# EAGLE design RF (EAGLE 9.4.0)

## Sheet 1 of 3: Board to Board Headers
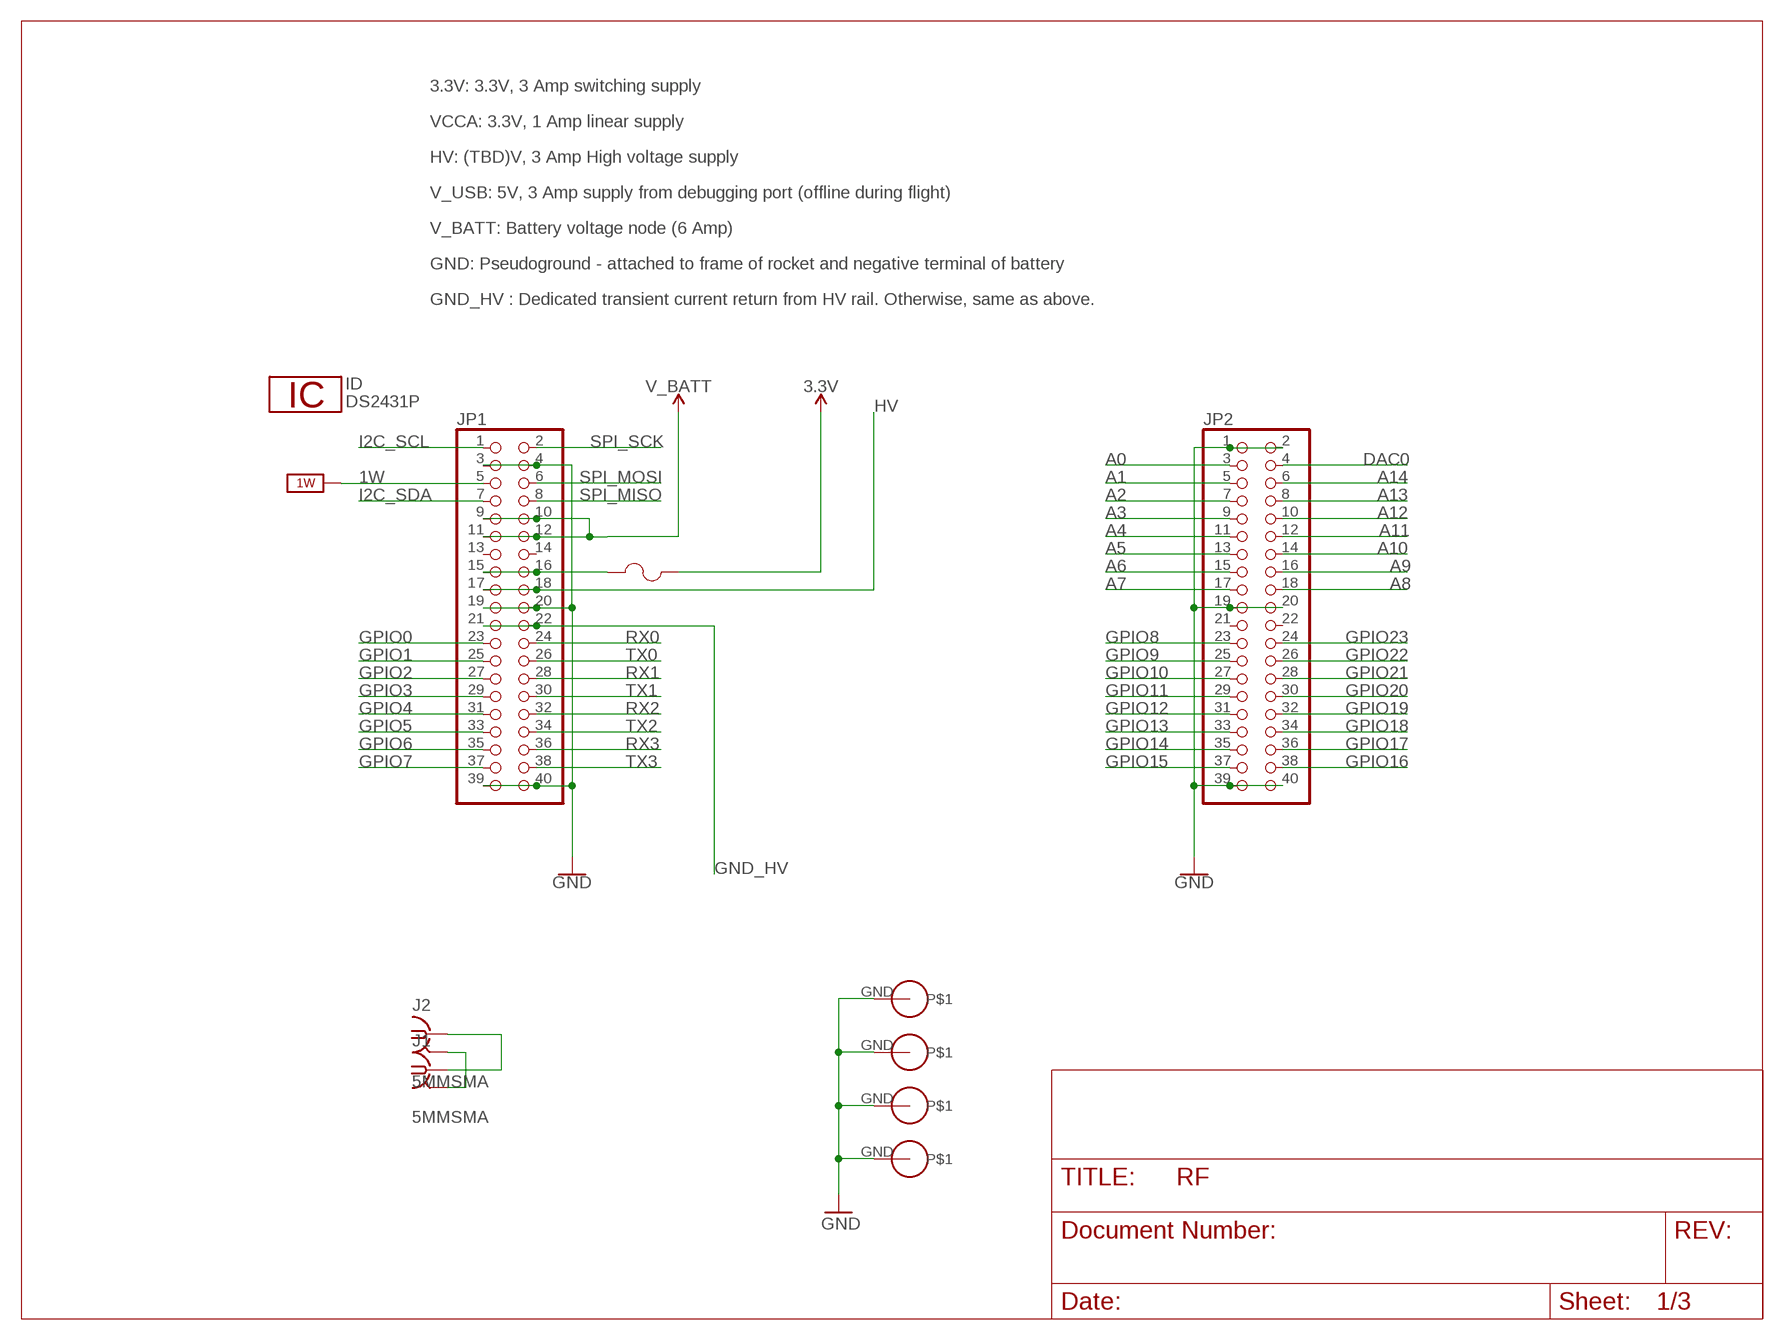
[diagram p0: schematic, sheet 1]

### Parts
F1  0603SFF150F/32-2  [FUS0603_TYCO]
ID  DS2431P  [TSOC6]
J1  5MMSMA  [5MMSMA]
J2  5MMSMA  [5MMSMA]
JP1  PINHD-2X20  [2X20]
JP2  PINHD-2X20  [2X20]
U$1  PS/104-MOUNTING-HOLE  [PC/104-MOUNTING-HOLE]
U$2  PS/104-MOUNTING-HOLE  [PC/104-MOUNTING-HOLE]
U$3  PS/104-MOUNTING-HOLE  [PC/104-MOUNTING-HOLE]
U$4  PS/104-MOUNTING-HOLE  [PC/104-MOUNTING-HOLE]

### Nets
1W: JP1.5 ; supply symbol labelled 1W_SUP
3.3V: F1.2 ; also sheet 2
A0: JP2.3
A1: JP2.5
A2: JP2.7
A3: JP2.9
A4: JP2.11
A5: JP2.13
A6: JP2.15
A7: JP2.17
A8: JP2.18
A9: JP2.16
A10: JP2.14
A11: JP2.12
A12: JP2.10
A13: JP2.8
A14: JP2.6
DAC0: JP2.4
GND: J1.GND J1.GND2(GND) J2.GND J2.GND2(GND) JP1.3 JP1.4 JP1.19 JP1.20 JP1.39 JP1.40 JP2.1 JP2.2 JP2.19 JP2.20 JP2.39 JP2.40 U$1.GND U$2.GND U$3.GND U$4.GND ; also sheet 2
GND_HV: JP1.21 JP1.22
GPIO0: JP1.23
GPIO1: JP1.25
GPIO2: JP1.27
GPIO3: JP1.29
GPIO4: JP1.31
GPIO5: JP1.33
GPIO6: JP1.35
GPIO7: JP1.37
GPIO8: JP2.23
GPIO9: JP2.25
GPIO10: JP2.27
GPIO11: JP2.29
GPIO12: JP2.31
GPIO13: JP2.33
GPIO14: JP2.35
GPIO15: JP2.37
GPIO16: JP2.38
GPIO17: JP2.36
GPIO18: JP2.34
GPIO19: JP2.32
GPIO20: JP2.30
GPIO21: JP2.28
GPIO22: JP2.26
GPIO23: JP2.24
HV: JP1.17 JP1.18
I2C_SCL: JP1.1
I2C_SDA: JP1.7
N$3: F1.1 JP1.15 JP1.16
N$4: JP1.9 JP1.10 JP1.11 JP1.12
N$8: J1.RF J2.RF
RX0: JP1.24 ; also sheet 2
RX1: JP1.28 ; also sheet 2
RX2: JP1.32 ; also sheet 2
RX3: JP1.36
SPI_MISO: JP1.8
SPI_MOSI: JP1.6
SPI_SCK: JP1.2
TX0: JP1.26 ; also sheet 2
TX1: JP1.30 ; also sheet 2
TX2: JP1.34 ; also sheet 2
TX3: JP1.38
Unconnected: JP1.13 JP1.14 JP2.21 JP2.22

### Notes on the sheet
- 3.3V: 3.3V, 3 Amp switching supply
- VCCA: 3.3V, 1 Amp linear supply
- HV: (TBD)V, 3 Amp High voltage supply
- V_USB: 5V, 3 Amp supply from debugging port (offline during flight)
- V_BATT: Battery voltage node (6 Amp)
- GND: Pseudoground - attached to frame of rocket and negative terminal of battery
- GND_HV : Dedicated transient current return from HV rail. Otherwise, same as above.

## Sheet 2 of 3: RN2483 434MHz RF module
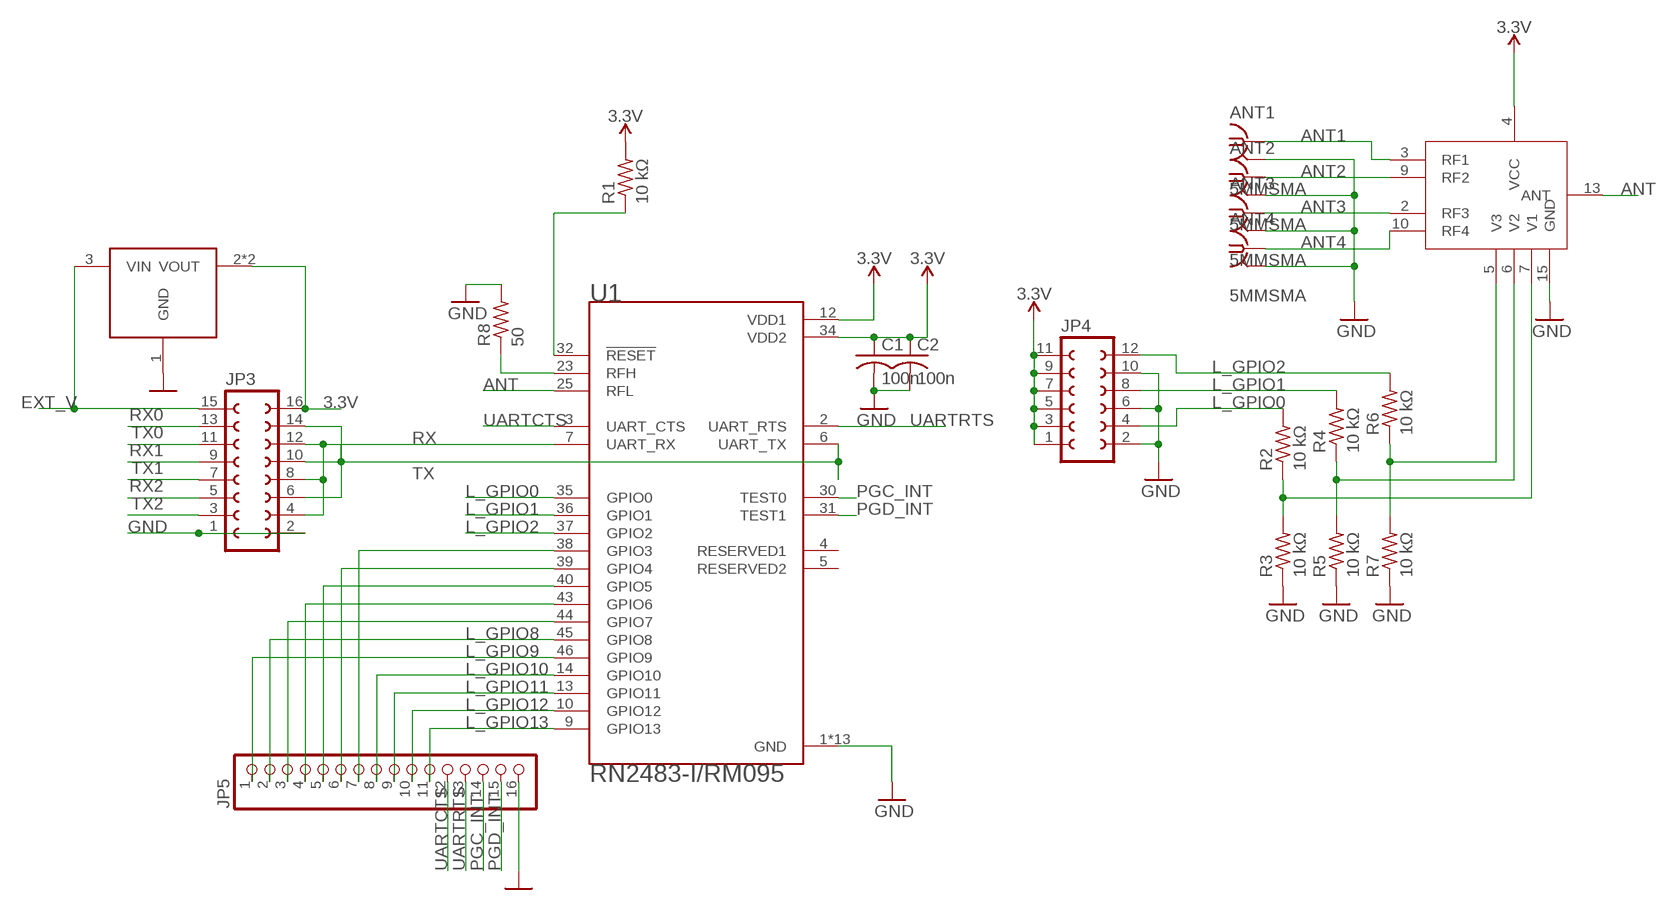
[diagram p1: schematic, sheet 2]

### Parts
ANT1  5MMSMA  [5MMSMA]
ANT2  5MMSMA  [5MMSMA]
ANT3  5MMSMA  [5MMSMA]
ANT4  5MMSMA  [5MMSMA]
C1  100n  C-USC0805  [C0805]
C2  100n  C-USC0805  [C0805]
JP3  FE08-2  [FE08-2]
JP4  FE06-2  [FE06-2]
JP5  PINHD-1X16  [1X16]
R1  10 kΩ  R-US_R1206  [R1206]
R2  10 kΩ  R-US_R1206  [R1206]
R3  10 kΩ  R-US_R1206  [R1206]
R4  10 kΩ  R-US_R1206  [R1206]
R5  10 kΩ  R-US_R1206  [R1206]
R6  10 kΩ  R-US_R1206  [R1206]
R7  10 kΩ  R-US_R1206  [R1206]
R8  50  R-US_R1206  [R1206]
U1  RN2483-I/RM095  [MICROCHIP_RN2483-I/RM095]
U2  SKY13414  [QFN45P200X200X55-15N]
U3  LDL1117S33R  [SOT223]

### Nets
3.3V: C1.1 C2.1 JP3.16 JP4.1 JP4.3 JP4.5 JP4.7 JP4.9 JP4.11 R1.2 U1.12(VDD1) U1.34(VDD2) U2.4(VCC) U3.2(VOUT) U3.4(VOUT) ; also sheet 1
ANT: U1.25(RFL) U2.13(ANT)
ANT1: ANT1.RF U2.3(RF1)
ANT2: ANT2.RF U2.9(RF2)
ANT3: ANT3.RF U2.2(RF3)
ANT4: ANT4.RF U2.10(RF4)
EXT_V: JP3.15 U3.3(VIN)
GND: ANT1.GND ANT1.GND2(GND) ANT2.GND ANT2.GND2(GND) ANT3.GND ANT3.GND2(GND) ANT4.GND ANT4.GND2(GND) C1.2 C2.2 JP3.1 JP3.2 JP4.2 JP4.6 JP4.10 JP5.16 R3.1 R5.1 R7.1 R8.2 U1.1(GND) U1.8(GND) U1.11(GND) U1.20(GND) U1.21(GND) U1.22(GND) U1.24(GND) U1.26(GND) U1.27(GND) U1.28(GND) U1.33(GND) U1.41(GND) U1.47(GND) U2.15(GND) U3.1(GND) ; also sheet 1
L_GPIO0: JP4.4 R2.2 U1.35(GPIO0)
L_GPIO1: JP4.8 R4.2 U1.36(GPIO1)
L_GPIO2: JP4.12 R6.2 U1.37(GPIO2)
L_GPIO8: JP5.2 U1.45(GPIO8)
L_GPIO9: JP5.1 U1.46(GPIO9)
L_GPIO10: JP5.8 U1.14(GPIO10)
L_GPIO11: JP5.9 U1.13(GPIO11)
L_GPIO12: JP5.10 U1.10(GPIO12)
L_GPIO13: JP5.11 U1.9(GPIO13)
N$1: R2.1 R3.2 U2.7(V1)
N$2: R4.1 R5.2 U2.6(V2)
N$7: R6.1 R7.2 U2.5(V3)
N$9: R1.1 U1.32(!RESET)
N$10: R8.1 U1.23(RFH)
N$16: JP5.3 U1.44(GPIO7)
N$17: JP5.4 U1.43(GPIO6)
N$18: JP5.5 U1.40(GPIO5)
N$19: JP5.6 U1.39(GPIO4)
N$20: JP5.7 U1.38(GPIO3)
PGC_INT: JP5.14 U1.30(TEST0)
PGD_INT: JP5.15 U1.31(TEST1)
RX: JP3.6 JP3.10 JP3.14 U1.6(UART_TX)
RX0: JP3.13 ; also sheet 1
RX1: JP3.9 ; also sheet 1
RX2: JP3.5 ; also sheet 1
TX: JP3.4 JP3.8 JP3.12 U1.7(UART_RX)
TX0: JP3.11 ; also sheet 1
TX1: JP3.7 ; also sheet 1
TX2: JP3.3 ; also sheet 1
UARTCTS: JP5.12 U1.3(UART_CTS)
UARTRTS: JP5.13 U1.2(UART_RTS)
Unconnected: U1.4(RESERVED1) U1.5(RESERVED2)

## Sheet 3 of 3: RN2903 903MHz RF module

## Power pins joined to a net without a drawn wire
1W: ID.2(1W)
GND: ID.1(GND)

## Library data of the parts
ANT1-ANT4 J1 J2 = CUINSPACE_Managed:5MMSMA
C1 C2 = rcl:C-US: CAPACITOR, American symbol; SPICEPREFIX: C
F1 = CU inSpace 2019 Parts:0603SFF150F/32-2; MANUFACTURER_PART_NUMBER: 0603SFF150F322; VENDOR: Littelfuse Inc
ID = 1wire:DS2431: 1024-Bit EEPROM
JP1 JP2 = pinhead:PINHD-2X20: PIN HEADER
JP3 = con-lsta:FE08-2: FEMALE HEADER; OC_FARNELL: unknown; OC_NEWARK: unknown
JP4 = con-lsta:FE06-2: FEMALE HEADER; OC_FARNELL: unknown; OC_NEWARK: unknown
JP5 = pinhead:PINHD-1X16: PIN HEADER
R1-R8 = rcl:R-US_: RESISTOR, American symbol; SPICEPREFIX: R
U1 = RN2483-I_RM095:RN2483-I/RM095: Sub-GHz Dual Band Long Range Transceiver LoRa Module; AVAILABILITY: Unavailable; DESCRIPTION: Sub-GHz Dual Band Long Range Transceiver LoRa Module; MF: Microchip; MP: RN2483-I/RM095; PACKAGE: None; PRICE: None
U2 = CUINSPACE_Managed:SKY13414
U3 = CUINSPACE_Managed:LDL1117S33R
U$1-U$4 = CU inSpace 2019 Parts:PS/104-MOUNTING-HOLE: Mounting hole for PC/104 board.

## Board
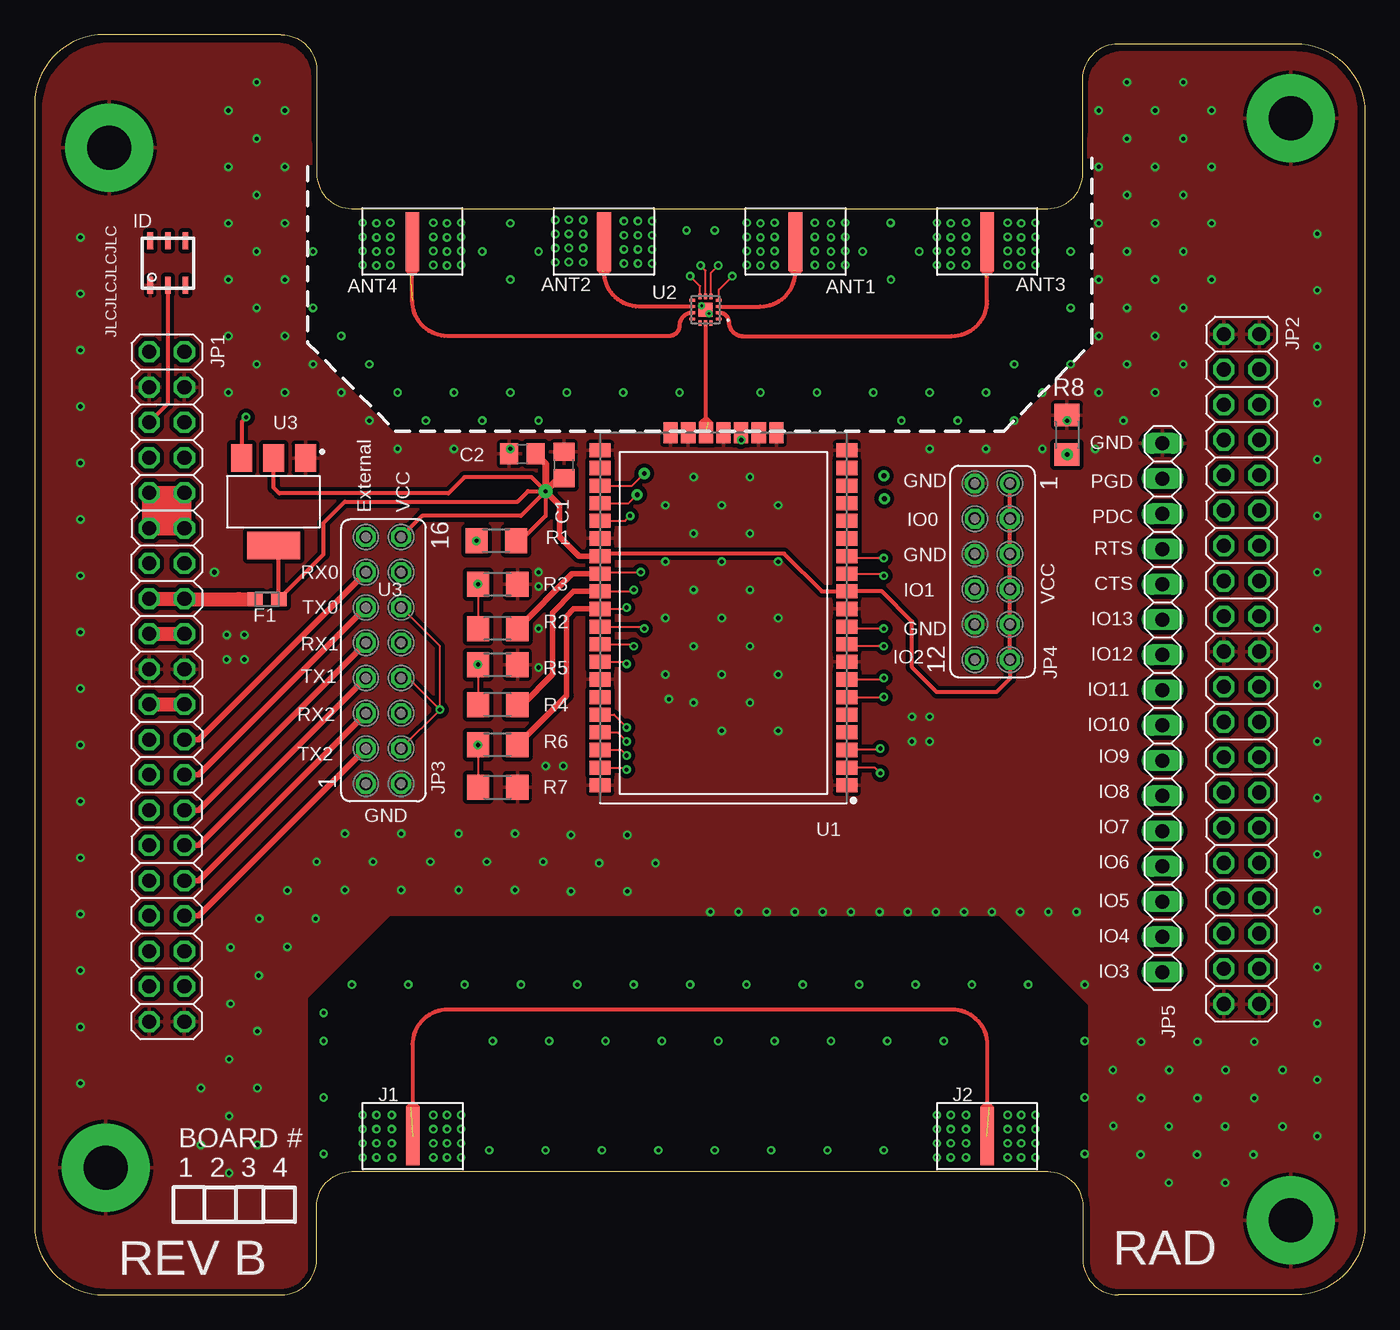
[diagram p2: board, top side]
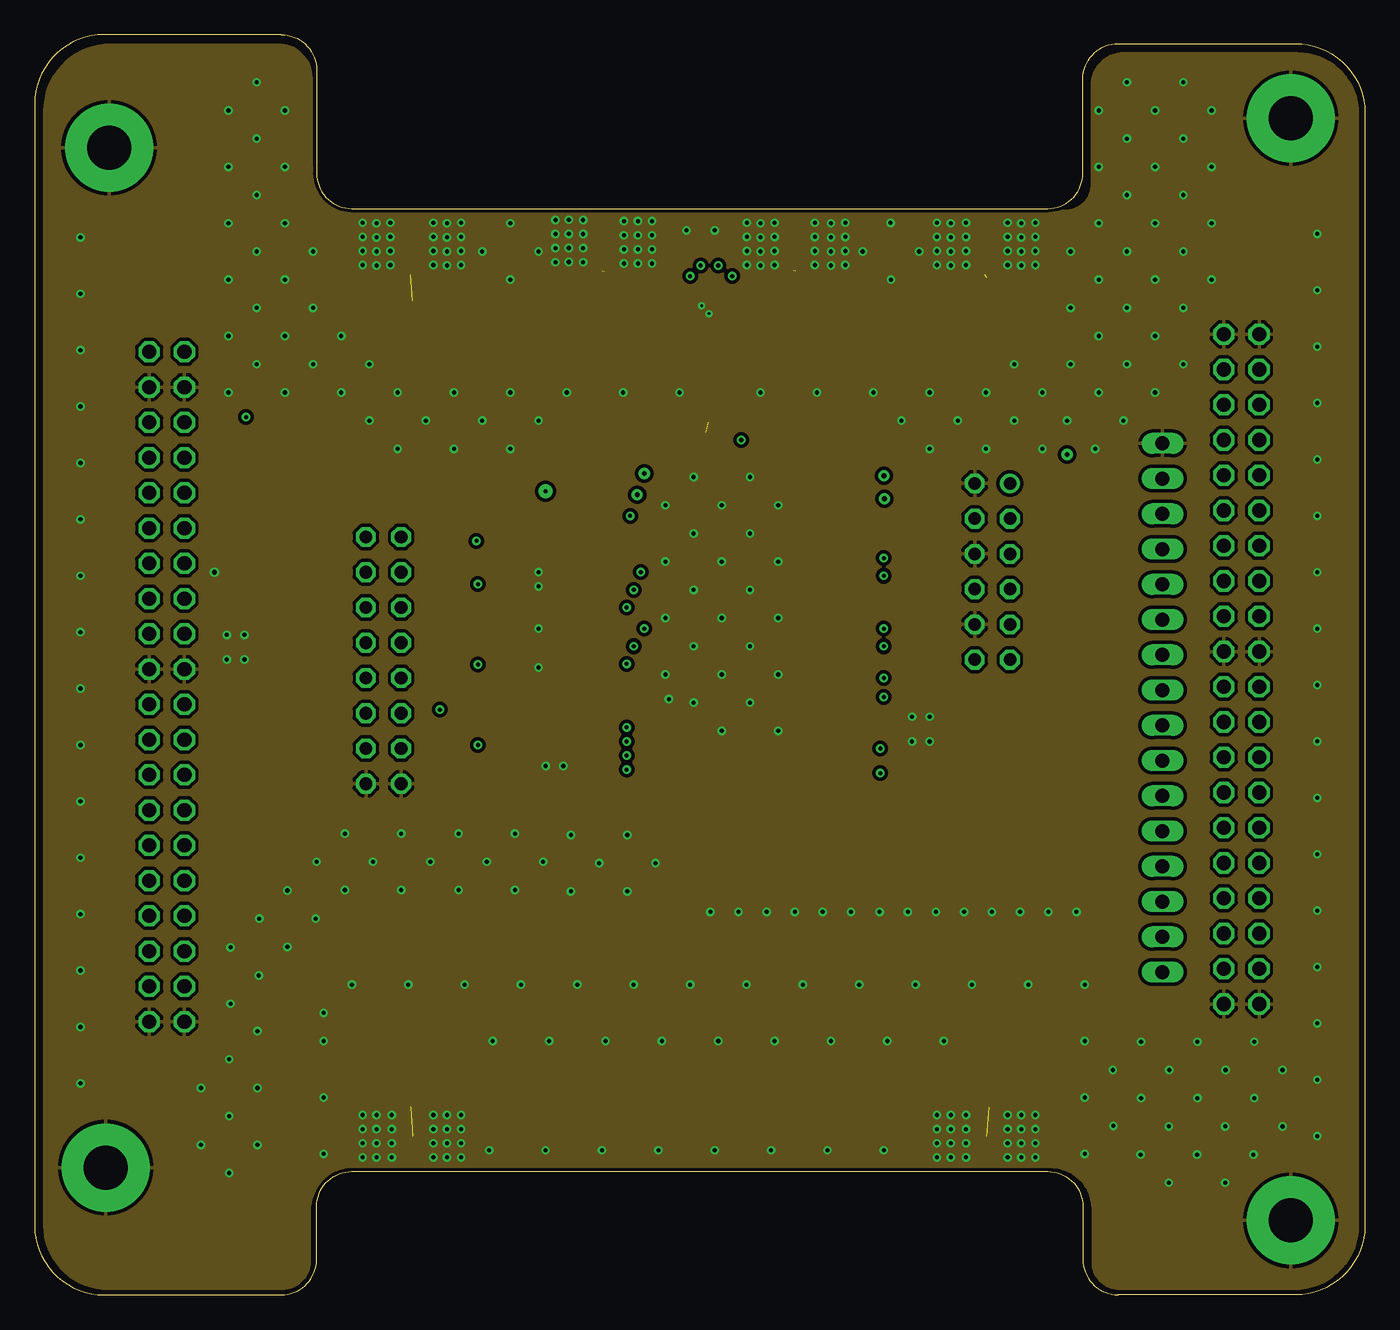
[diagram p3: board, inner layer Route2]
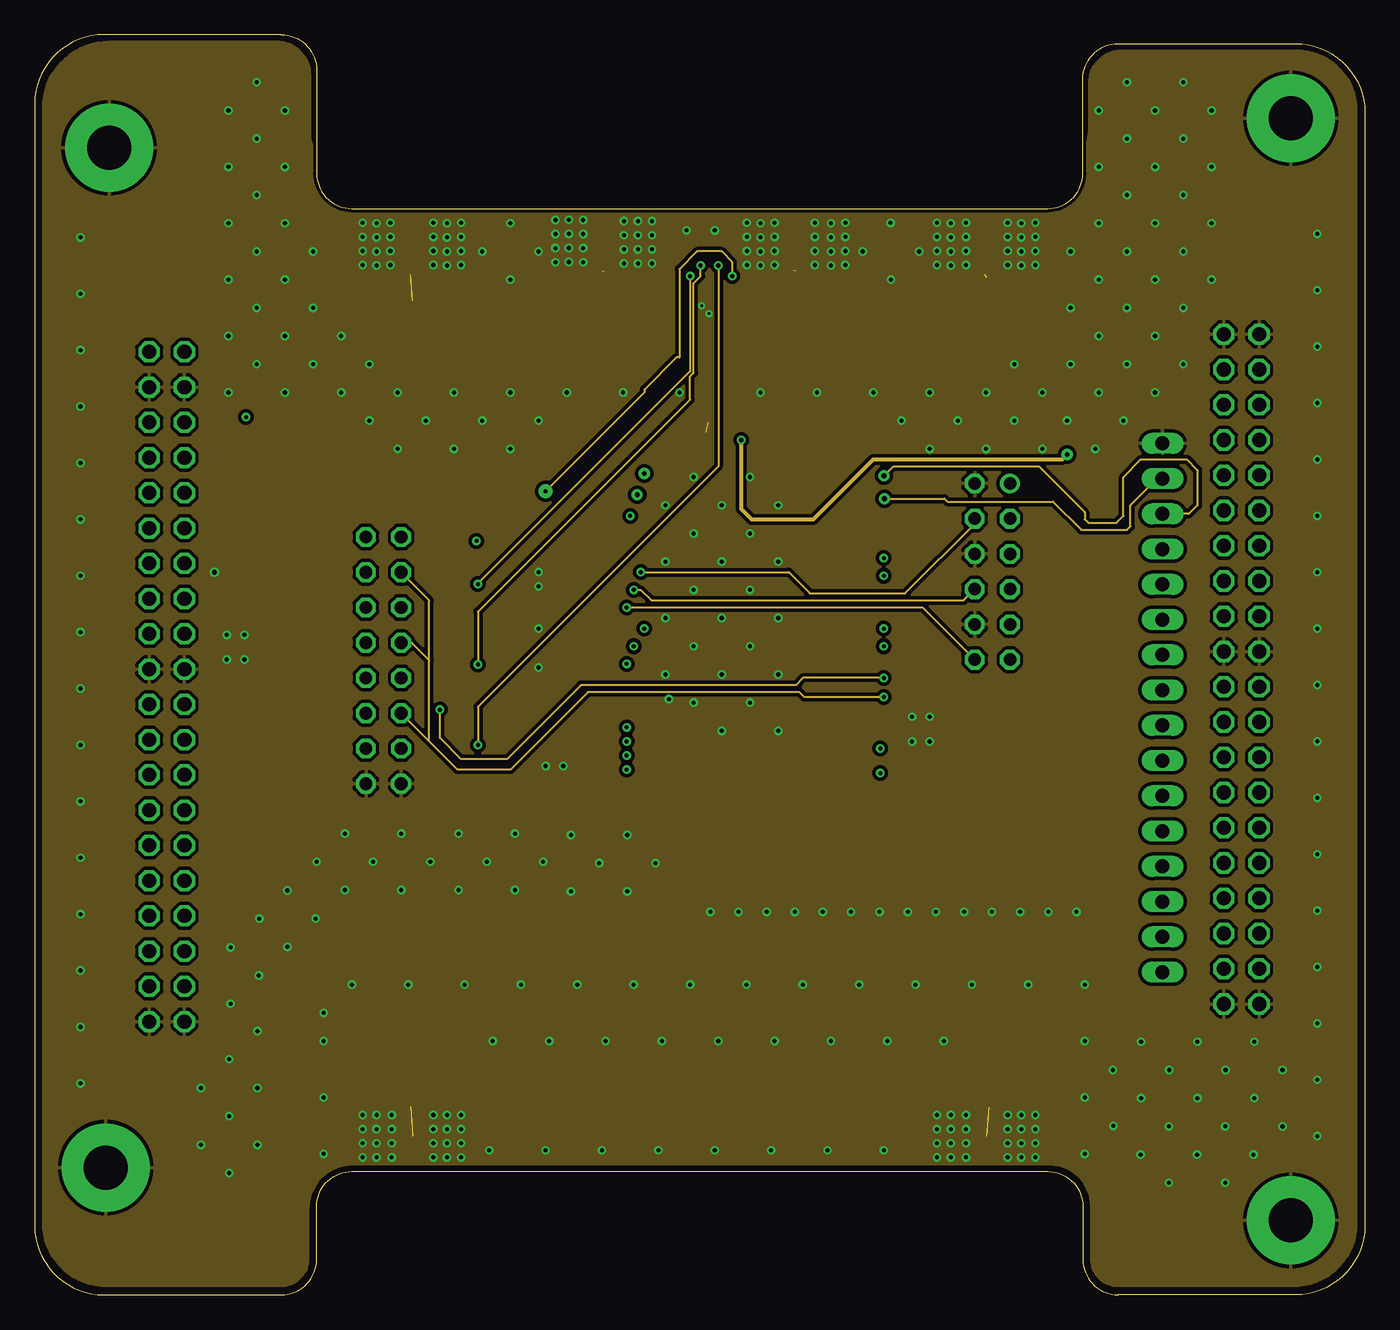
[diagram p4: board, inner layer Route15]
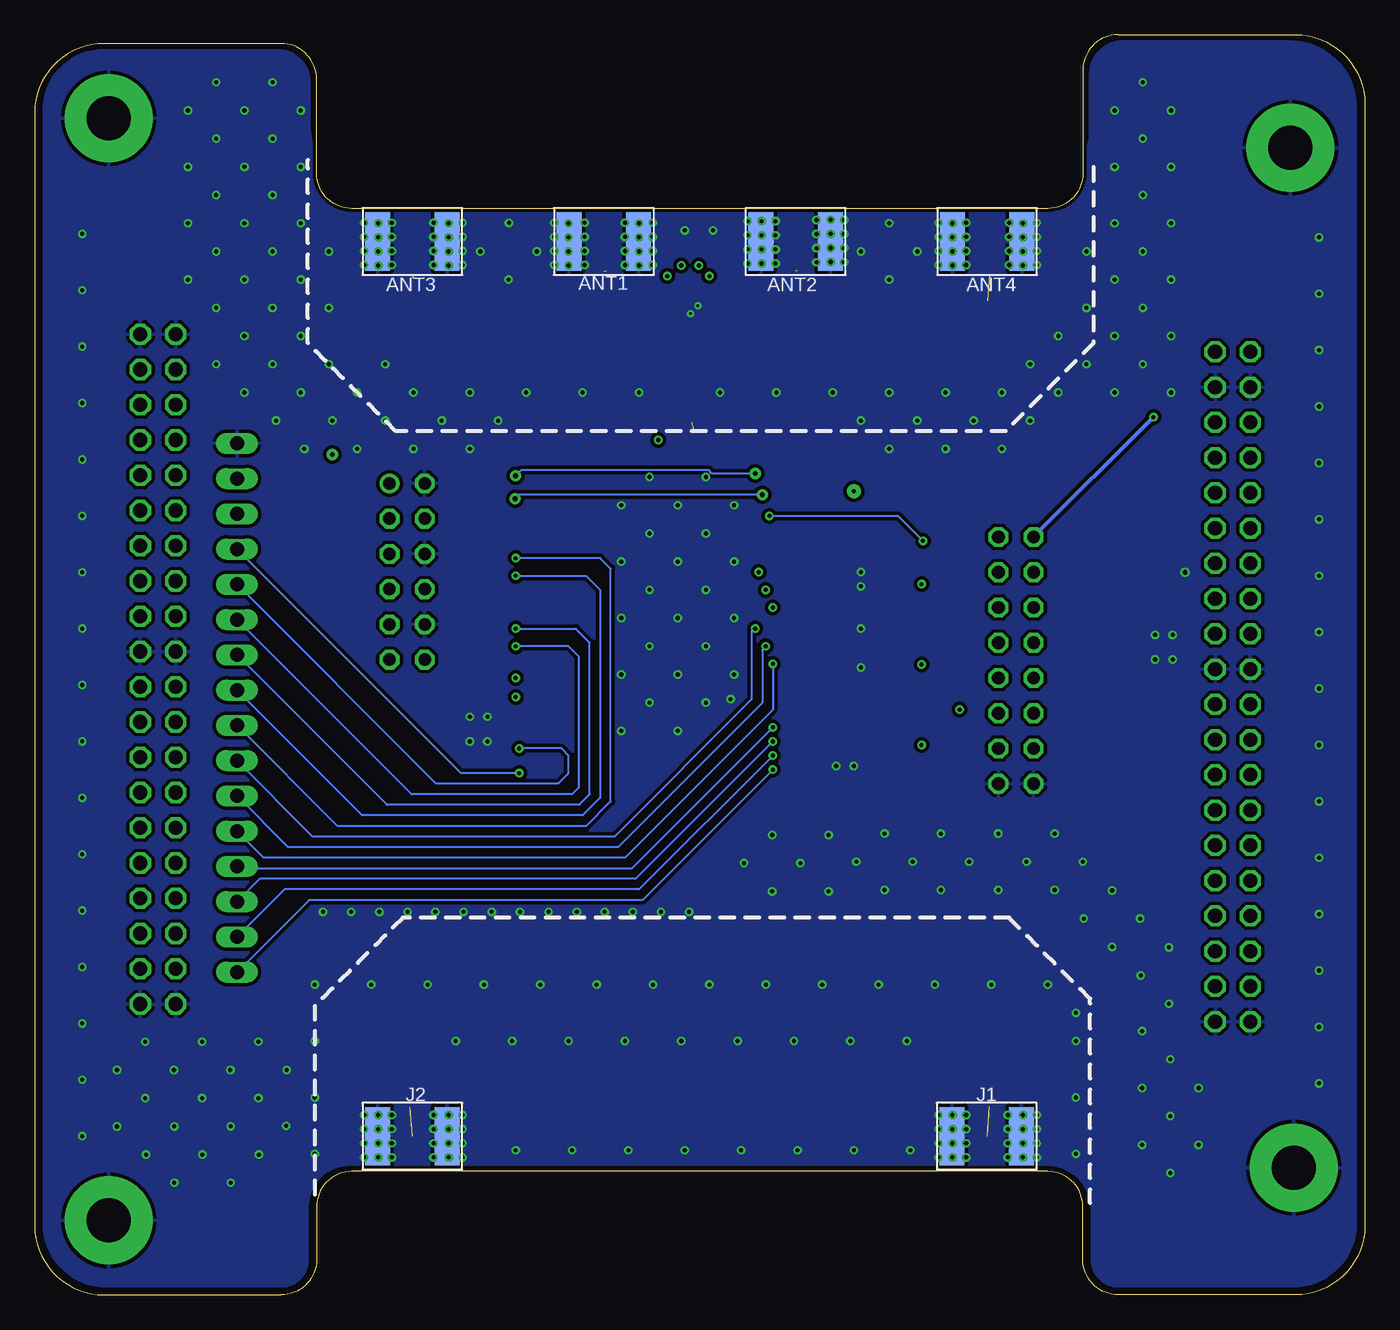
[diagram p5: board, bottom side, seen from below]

Size 95.89 x 90.81 mm. Coordinates in mm from the lower left corner, seen from the top.
Outline: 0,85.81 0,5 arc90 5,0 17.78,0 arc90 20.32,2.54 20.32,6.35 arc-90 22.86,8.89 73.03,8.89 arc-90 75.56,6.35 75.56,2.54 arc90 78.11,0 90.89,0 arc90 95.89,5 95.89,85.17 arc90 90.89,90.17 78.11,90.17 arc90 75.56,87.63 75.56,80.82 arc-90 73.03,78.28 22.86,78.28 arc-90 20.32,80.82 20.32,88.27 arc90 17.78,90.81 5,90.81 arc90 0,85.81
Copper layers (1+2*15+16): Top 0.035mm / dielectric 0.2mm / Route2 0.0175mm / dielectric 1.065mm / Route15 0.0175mm / dielectric 0.2mm / Bottom 0.035mm
Design rules "dirt_cheap_dirty_boards.v1 *": minimum track width 5mil, minimum drill 0.2mm, track to track 5mil, track to pad 5mil, pad to pad 5mil, via to via 5mil, smd to smd 0mil, copper to edge 10mil, drill to drill 10mil, minimum pad ring 10mil, minimum via ring 6mil, stop-mask expansion 2mil, vias tented up to drill 25mil, thermal gap 10mil

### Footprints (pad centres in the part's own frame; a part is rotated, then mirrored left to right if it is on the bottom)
5MMSMA = smd 1.8 x 4.2 bottom: GND 2.5,0; GND2 -2.5,0 | smd 1 x 4.2: RF 0,0
C0805 = smd 1.3 x 1.5: 1 -0.95,0; 2 0.95,0
FUS0603_TYCO = smd 1.092 x 0.991: 1 -0.851,0; 2 0.851,0
TSOC6 = smd 0.406 x 1.219: 1 -1.27,-1.6; 2 0,-1.6; 3 1.27,-1.6; 4 1.27,1.6; 5 0,1.6; 6 -1.27,1.6
2X20 = drill 1.016 octagon: 1 -24.13,-1.27; 2 -24.13,1.27; 3 -21.59,-1.27; 4 -21.59,1.27; 5 -19.05,-1.27; 6 -19.05,1.27; 7 -16.51,-1.27; 8 -16.51,1.27; 9 -13.97,-1.27; 10 -13.97,1.27; 11 -11.43,-1.27; 12 -11.43,1.27; 13 -8.89,-1.27; 14 -8.89,1.27; 15 -6.35,-1.27; 16 -6.35,1.27; 17 -3.81,-1.27; 18 -3.81,1.27; 19 -1.27,-1.27; 20 -1.27,1.27; 21 1.27,-1.27; 22 1.27,1.27; 23 3.81,-1.27; 24 3.81,1.27; 25 6.35,-1.27; 26 6.35,1.27; 27 8.89,-1.27; 28 8.89,1.27; 29 11.43,-1.27; 30 11.43,1.27; 31 13.97,-1.27; 32 13.97,1.27; 33 16.51,-1.27; 34 16.51,1.27; 35 19.05,-1.27; 36 19.05,1.27; 37 21.59,-1.27; 38 21.59,1.27; 39 24.13,-1.27; 40 24.13,1.27
FE08-2 = drill 0.914 octagon: 1 -8.89,1.27; 2 -8.89,-1.27; 3 -6.35,1.27; 4 -6.35,-1.27; 5 -3.81,1.27; 6 -3.81,-1.27; 7 -1.27,1.27; 8 -1.27,-1.27; 9 1.27,1.27; 10 1.27,-1.27; 11 3.81,1.27; 12 3.81,-1.27; 13 6.35,1.27; 14 6.35,-1.27; 15 8.89,1.27; 16 8.89,-1.27
FE06-2 = drill 0.914: 1 -6.35,1.27 | drill 0.914 octagon: 2 -6.35,-1.27; 3 -3.81,1.27; 4 -3.81,-1.27; 5 -1.27,1.27; 6 -1.27,-1.27; 7 1.27,1.27; 8 1.27,-1.27; 9 3.81,1.27; 10 3.81,-1.27; 11 6.35,1.27; 12 6.35,-1.27
1X16 = drill 1.016 long: 1 -19.05,0; 2 -16.51,0; 3 -13.97,0; 4 -11.43,0; 5 -8.89,0; 6 -6.35,0; 7 -3.81,0; 8 -1.27,0; 9 1.27,0; 10 3.81,0; 11 6.35,0; 12 8.89,0; 13 11.43,0; 14 13.97,0; 15 16.51,0; 16 19.05,0
R1206 = smd 1.6 x 1.803: 1 -1.422,0; 2 1.422,0
MICROCHIP_RN2483-I/RM095 = smd 1.524 x 1.016: 1 -8.89,12.065; 2 -8.89,10.795; 3 -8.89,9.525; 4 -8.89,8.255; 5 -8.89,6.985; 6 -8.89,5.715; 7 -8.89,4.445; 8 -8.89,3.175; 9 -8.89,1.905; 10 -8.89,0.635; 11 -8.89,-0.635; 12 -8.89,-1.905; 13 -8.89,-3.175; 14 -8.89,-4.445; 15 -8.89,-5.715; 16 -8.89,-6.985; 17 -8.89,-8.255; 18 -8.89,-9.525; 19 -8.89,-10.795; 20 -8.89,-12.065; 28 8.89,-12.065; 29 8.89,-10.795; 30 8.89,-9.525; 31 8.89,-8.255; 32 8.89,-6.985; 33 8.89,-5.715; 34 8.89,-4.445; 35 8.89,-3.175; 36 8.89,-1.905; 37 8.89,-0.635; 38 8.89,0.635; 39 8.89,1.905; 40 8.89,3.175; 41 8.89,4.445; 42 8.89,5.715; 43 8.89,6.985; 44 8.89,8.255; 45 8.89,9.525; 46 8.89,10.795; 47 8.89,12.065 | smd 1.016 x 1.524: 21 -3.81,-13.335; 22 -2.54,-13.335; 23 -1.27,-13.335; 24 0,-13.335; 25 1.27,-13.335; 26 2.54,-13.335; 27 3.81,-13.335
QFN45P200X200X55-15N = smd 0.2 x 0.395: 1 -0.675,-0.953; 2 -0.225,-0.953; 3 0.225,-0.953; 4 0.675,-0.953; 8 0.675,0.953; 9 0.225,0.953; 10 -0.225,0.953; 11 -0.675,0.953 | smd 0.395 x 0.2: 5 0.953,-0.4; 6 0.953,0; 7 0.953,0.4; 12 -0.953,0.4; 13 -0.953,0; 14 -0.953,-0.4 | smd 1 x 1: 15 0,0
SOT223 = smd 1.5 x 2: 1 -2.3,-3.15; 2 0,-3.15; 3 2.3,-3.15 | smd 3.8 x 2: 4 0,3.15
PC/104-MOUNTING-HOLE = drill 3.175 pad 6.35: GND 0,0

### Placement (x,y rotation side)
ANT1  54.85,75.9 180 top
ANT2  41.04,75.9 0 top
ANT3  68.66,75.9 0 top
ANT4  27.22,75.9 0 top
C1  38.15,59.79 90 top
C2  35.15,60.6 180 top
F1  16.75,50.13 0 top
ID  9.6,74.35 0 top
J1  27.26,11.43 0 top
J2  68.66,11.43 0 top
JP1  9.53,43.81 270 top
JP2  87,45.09 270 top
JP3  25.15,45.72 90 top
JP4  69.04,52.12 270 top
JP5  81.3,42.3 90 top
R1  33.27,54.33 0 top
R2  33.38,48.01 0 top
R3  33.38,51.21 180 top
R4  33.38,42.52 0 top
R5  33.38,45.42 180 top
R6  33.38,39.62 0 top
R7  33.38,36.58 180 top
R8  74.42,61.98 90 top
U1  49.65,48.79 180 top
U2  48.36,70.99 90 top
U3  17.22,57.15 180 top
U$1  5.36,82.65 0 top
U$2  90.55,84.79 0 top
U$3  5.13,9.17 0 top
U$4  90.55,5.36 0 top

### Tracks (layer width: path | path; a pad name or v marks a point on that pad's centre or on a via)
1W
  Top 0.305: ID.2 9.6,64.21 JP1.5
3.3V  (via drill 0.3 pad 0.45, 0.3 pad 1)
  Top 0.127: U2.4 49.31,72.43 v50.29,73.41
  Top 0.305: 17.6,53.62 F1.2 20.83,53.35 20.83,55.63 22.35,57.15 34.8,57.15 35.56,57.91 v36.83,57.91 | U3.2 17.22,58.17 17.63,57.76 29.82,57.76 30.99,58.93 35.81,58.93 v36.83,57.91 | v36.83,57.91 35.05,56.13 27.94,56.13 JP3.16 | v36.83,57.91 36.83,56.13 35.11,54.42 34.78,54.42 | U1.34 40.94,53.41 54.03,53.41 56.75,50.69 U1.12 61.07,50.69 63.25,48.51 63.25,45.21 65.02,43.43 69.34,43.43 70.31,44.4 JP4.11 JP4.9 JP4.7 JP4.5 JP4.3 JP4.1 70.65,58.81
  Top 0.406: v36.83,57.91 37.85,56.9 37.85,54.61 39.22,53.23 U1.34 | 34.78,54.42 R1.2
  Top 0.508: C2.1 36.83,59.87 v36.83,57.91 37.76,58.84 C1.1
  Top 1.016: 17.6,53.62 U3.4
  Route15 0.127: v50.29,73.41 50.29,74.42 49.53,75.18 47.75,75.18 46.48,73.91 46.48,67.56 46.47,67.55 46.28,67.55 43.96,65.23 43.96,65.04 v36.83,57.91
ANT  (1 unrouted)
  Top 0.102: 48.84,62.88 48.54,63.18 48.24,63.18 48.04,62.98 | 48.04,62.98 47.94,62.88 48.24,62.88 48.24,63.08 48.14,62.98 | 48.14,62.98 48.04,62.98 | 48.14,62.98 48.54,62.98 48.54,63.08 48.64,62.98 | 48.64,62.98 48.74,62.88 48.54,62.88 48.64,62.98
  Top 0.293: U1.25 arc-90 48.36,62.14 U2.13
ANT1  (1 unrouted)
  Top 0.102: 54.4,73.8 54.7,73.5 55,73.5 55.2,73.7 | 55.2,73.7 55.3,73.8 55,73.8 55,73.6 55.1,73.7 | 55.1,73.7 55.2,73.7 | 55.1,73.7 54.7,73.7 54.7,73.6 54.6,73.7 | 54.6,73.7 54.5,73.8 54.7,73.8 54.6,73.7
  Top 0.293: U2.3 52.31,71.22 arc90 54.85,73.76 ANT1.RF
ANT2  (1 unrouted)
  Top 0.102: 40.6,73.8 40.9,73.5 41.2,73.5 41.4,73.7 | 41.4,73.7 41.5,73.8 41.2,73.8 41.2,73.6 41.3,73.7 | 41.3,73.7 41.4,73.7 | 41.3,73.7 40.9,73.7 40.9,73.6 40.8,73.7 | 40.8,73.7 40.7,73.8 40.9,73.8 40.8,73.7
  Top 0.293: U2.9 43.58,71.22 arc-90 41.04,73.76 ANT2.RF
ANT3  (1 unrouted)
  Top 0.102: 68.2,73.8 68.5,73.5 68.8,73.5 69,73.7 | 69,73.7 69.1,73.8 68.8,73.8 68.8,73.6 68.9,73.7 | 68.9,73.7 69,73.7 | 68.9,73.7 68.5,73.7 68.5,73.6 68.4,73.7 | 68.4,73.7 68.3,73.8 68.5,73.8 68.4,73.7
  Top 0.293: U2.2 49.37,70.77 arc-90 50.04,70.1 arc90 51.05,69.09 66.12,69.09 arc90 68.66,71.63 68.66,73.3 ANT3.RF
ANT4  (1 unrouted)
  Top 0.102: 26.77,73.81 27.07,73.51 27.37,73.51 27.57,73.71 | 27.57,73.71 27.67,73.81 27.37,73.81 27.37,73.61 27.47,73.71 | 27.47,73.71 27.57,73.71 | 27.47,73.71 27.07,73.71 27.07,73.61 26.97,73.71 | 26.97,73.71 26.87,73.81 27.07,73.81 26.97,73.71
  Top 0.293: U2.10 U2.10 arc90 46.48,69.85 arc-90 45.72,69.09 43.69,69.09 38.5,69.09 38.1,69.09 29.76,69.09 arc-90 27.22,71.63 ANT4.RF
EXT_V  (via drill 0.3 pad 0.45)
  Top 0.305: v15.24,63.25 14.92,62.93 U3.3
  Bottom 0.305: JP3.15 v15.24,63.25
GND  (via drill 0.2 pad 0.45, 0.3 pad 0.45, 0.35)
  Top 0.127: U2.15 48.62,70.74 v48.62,70.71
  other vias: 12.95,52.07 24.64,77.22 24.64,76.2 24.64,75.18 24.64,74.17 29.72,77.22 29.72,76.2 29.72,75.18 29.72,74.17 30.23,65.02 24.13,67.06 38.35,65.02 42.42,65.02 46.48,65.02 52.32,65.02 56.39,65.02 60.45,65.02 64.52,65.02 68.58,65.02 70.61,67.06 13.97,65.02 16,67.06 18.03,65.02 20.07,67.06 22.1,65.02 13.97,69.09 16,71.12 18.03,69.09 20.07,71.12 22.1,69.09 13.97,73.15 16,75.18 18.03,73.15 20.07,75.18 34.29,65.02 26.16,65.02 13.97,77.22 16,79.25 18.03,77.22 13.97,81.28 16,83.31 18.03,81.28 13.97,85.34 16,87.38 18.03,85.34 32.26,75.18 34.29,77.22 36.32,75.18 61.7,77.24 59.69,75.18 63.75,75.18 80.77,77.22 82.8,79.25 84.84,77.22 80.77,81.28 82.8,83.31 84.84,81.28 80.77,85.34 82.8,87.38 84.84,85.34 80.77,65.02 82.8,67.06 80.77,69.09 82.8,71.12 80.77,73.15 82.8,75.18 84.84,73.15 74.68,67.06 76.71,65.02 78.74,67.06 74.68,71.12 76.71,69.09 78.74,71.12 74.68,75.18 76.71,73.15 78.74,75.18 76.71,77.22 78.74,79.25 76.71,81.28 78.74,83.31 76.71,85.34 78.74,87.38 74.42,62.99 76.45,60.96 78.49,62.99 68.58,60.96 70.61,62.99 72.64,60.96 62.48,62.99 64.52,60.96 66.55,62.99 32.26,62.99 24.13,62.99 26.16,60.96 30.23,60.96 28.19,62.99 45.47,56.9 47.5,58.93 49.53,56.9 51.56,58.93 53.59,56.9 45.47,52.83 47.5,54.86 49.53,52.83 51.56,54.86 53.59,52.83 45.47,48.77 47.5,50.8 49.53,48.77 51.56,50.8 53.59,48.77 45.47,44.7 47.5,46.74 49.53,44.7 51.56,46.74 53.59,44.7 45.72,42.93 47.5,42.67 49.53,40.64 51.56,42.67 53.59,40.64 48.08,71.27 22.86,22.35 26.92,22.35 30.99,22.35 35.05,22.35 39.12,22.35 20.83,10.16 20.83,14.22 20.83,20.32 20.83,18.29 33.02,18.29 37.08,18.29 41.15,18.29 45.21,18.29 49.28,18.29 53.34,18.29 57.4,18.29 61.47,18.29 65.53,18.29 75.69,18.29 47.24,22.35 43.18,22.35 51.31,22.35 55.37,22.35 59.44,22.35 63.5,22.35 67.56,22.35 71.63,22.35 75.69,22.35 75.69,14.22 75.69,10.16 40.89,10.41 36.83,10.41 44.96,10.41 49.02,10.41 53.09,10.41 57.15,10.41 61.21,10.41 32.77,10.41 24.64,12.95 24.64,11.94 24.64,10.92 24.64,9.91 29.72,12.95 29.72,11.94 29.72,10.92 29.72,9.91 66.04,12.95 66.04,11.94 66.04,10.92 66.04,9.91 71.12,12.95 71.12,11.94 71.12,10.92 71.12,9.91 38.51,77.47 38.51,76.45 38.51,75.44 38.51,74.42 43.49,77.37 43.49,76.35 43.49,75.34 43.49,74.32 52.32,77.22 52.32,76.2 52.32,75.18 52.32,74.17 57.4,77.22 57.4,76.2 57.4,75.18 57.4,74.17 66.04,77.22 66.04,76.2 66.04,75.18 66.04,74.17 71.12,77.22 71.12,76.2 71.12,75.18 71.12,74.17 36.83,38.1 38.1,38.1 36.32,45.21 36.32,48.01 36.32,51.05 36.32,52.07 72.64,65.02 92.46,48.01 92.46,52.07 92.46,56.13 92.46,64.26 92.46,60.2 92.46,68.33 92.46,72.39 92.46,76.45 92.46,11.43 92.46,15.49 92.46,19.56 92.46,27.69 92.46,23.62 92.46,31.75 92.46,35.81 92.46,39.88 92.46,43.94 64.52,41.66 63.25,41.66 64.52,39.88 63.25,39.88 3.3,15.24 3.3,19.3 3.3,23.37 3.3,31.5 3.3,27.43 3.3,35.56 3.3,39.62 3.3,43.69 3.3,47.75 3.3,51.82 3.3,55.88 3.3,59.94 3.3,68.07 3.3,64.01 3.3,72.14 3.3,76.2 36.32,62.99 34.29,60.96 23.64,77.25 23.64,76.24 23.64,75.22 23.64,74.21 25.64,77.25 25.64,76.24 25.64,75.22 25.64,74.21 28.74,77.25 28.74,76.24 28.74,75.22 28.74,74.21 30.74,77.25 30.74,76.24 30.74,75.22 30.74,74.21 37.54,77.45 37.54,76.44 37.54,75.42 37.54,74.41 39.54,77.45 39.54,76.44 39.54,75.42 39.54,74.41 51.34,77.25 51.34,76.24 51.34,75.22 51.34,74.21 53.34,77.25 53.34,76.24 53.34,75.22 53.34,74.21 56.24,77.25 56.24,76.24 56.24,75.22 56.24,74.21 58.44,77.25 58.44,76.24 58.44,75.22 58.44,74.21 65.04,77.25 65.04,76.24 65.04,75.22 65.04,74.21 67.14,77.25 67.14,76.24 67.14,75.22 67.14,74.21 70.14,77.25 70.14,76.24 70.14,75.22 70.14,74.21 72.14,77.25 72.14,76.24 72.14,75.22 72.14,74.21 42.47,77.37 42.47,76.35 42.47,75.34 42.47,74.32 44.5,77.37 44.5,76.35 44.5,75.34 44.5,74.32 49.02,76.71 46.99,76.71 34.29,73.15 61.72,73.15 23.64,12.95 23.64,11.94 23.64,10.92 23.64,9.91 25.74,12.95 25.74,11.94 25.74,10.92 25.74,9.91 28.74,12.95 28.74,11.94 28.74,10.92 28.74,9.91 30.74,12.95 30.74,11.94 30.74,10.92 30.74,9.91 65.04,12.95 65.04,11.94 65.04,10.92 65.04,9.91 67.14,12.95 67.14,11.94 67.14,10.92 67.14,9.91 70.14,12.95 70.14,11.94 70.14,10.92 70.14,9.91 72.14,12.95 72.14,11.94 72.14,10.92 72.14,9.91 60.91,27.6 62.94,27.6 64.97,27.6 67,27.6 69.01,27.6 71.04,27.6 73.07,27.6 75.1,27.6 56.81,27.6 58.84,27.6 48.71,27.6 50.74,27.6 52.77,27.6 54.8,27.6 44.75,31.1 42.72,29.07 40.69,31.1 42.72,33.14 38.66,29.07 38.66,33.14 36.65,31.2 34.62,29.17 32.59,31.2 34.62,33.24 30.56,29.17 28.52,31.2 30.56,33.24 26.42,29.17 24.39,31.2 26.42,33.24 22.36,29.17 20.32,31.2 22.36,33.24 20.25,27.1 18.22,25.07 16.19,27.1 18.22,29.14 16.15,23 14.12,20.97 14.12,25.04 16.05,19 14.02,16.97 16.05,14.9 14.02,12.87 11.99,14.9 16.05,10.8 14.02,8.77 11.99,10.8 15.12,47.56 13.85,47.56 15.12,45.78 13.85,45.78 77.76,12.17 85.85,16.2 83.82,14.17 81.79,16.2 83.82,18.24 79.76,14.17 77.72,16.2 79.76,18.24 87.85,10.1 85.82,8.07 83.79,10.1 85.82,12.14 81.76,8.07 79.72,10.1 81.76,12.14 89.95,16.2 87.92,14.17 87.92,18.24 89.96,12.13
  pour Top (isolate 0.305, rank 3): 19.81,87.79 19.81,83.5 arc90 22.41,80.9 73.1,80.9 arc90 76.05,83.85 76.05,87.19 arc-90 78.4,89.53 90.92,89.53 arc-90 95.25,85.21 95.25,5.04 arc-90 90.72,0.51 78.11,0.51 arc-90 76.2,2.41 76.2,6.25 arc90 73.18,9.27 22.91,9.27 arc90 19.68,6.05 19.68,2.45 arc-90 17.74,0.51 5.19,0.51 arc-90 0.64,5.06 0.64,85.4 arc-90 5.4,90.17 17.43,90.17 arc-90
  pour Bottom (isolate 0.254): 19.81,87.92 19.81,83.63 arc90 22.41,81.03 73.1,81.03 arc90 76.05,83.98 76.05,87.31 arc-90 78.4,89.66 90.92,89.66 arc-90 95.25,85.33 95.25,5.17 arc-90 90.72,0.64 78.11,0.64 arc-90 76.2,2.54 76.2,6.38 arc90 73.18,9.4 22.91,9.4 arc90 19.68,6.17 19.68,2.58 arc-90 17.74,0.64 5.19,0.64 arc-90 0.64,5.19 0.64,85.53 arc-90 5.4,90.3 17.43,90.3 arc-90
  pour Route15 (isolate 0.254): 19.81,87.92 19.81,83.63 arc90 22.41,81.03 73.1,81.03 arc90 76.05,83.98 76.05,87.31 arc-90 78.4,89.66 90.92,89.66 arc-90 95.25,85.33 95.25,5.17 arc-90 90.72,0.64 78.11,0.64 arc-90 76.2,2.54 76.2,6.38 arc90 73.18,9.4 22.91,9.4 arc90 19.68,6.17 19.68,2.58 arc-90 17.74,0.64 5.19,0.64 arc-90 0.64,5.19 0.64,85.53 arc-90 5.4,90.3 17.43,90.3 arc-90
  pour Route2 (isolate 0.254): 19.91,87.72 19.91,81.93 arc90 23.71,78.13 74.3,78.13 arc90 76.25,80.08 76.25,87.21 arc-90 78.5,89.46 91.02,89.46 arc-90 95.35,85.13 95.35,4.97 arc-90 90.82,0.43 78.2,0.43 arc-90 76.3,2.34 76.3,6.18 arc90 73.28,9.2 23.01,9.2 arc90 19.79,5.97 19.79,2.38 arc-90 17.84,0.43 5.29,0.43 arc-90 0.73,4.99 0.73,85.33 arc-90 5.5,90.1 17.53,90.1 arc-90
GND_HV
  Top 1.016: JP1.21 JP1.22
HV
  Top 1.016: JP1.17 JP1.18
KEEPOUT
  cutout Top (no thermals): 19.68,81.28 19.68,68.58 26.04,62.23 69.85,62.23 76.2,68.58 76.2,81.92 75.56,81.28
KEEPOUT1
  cutout Top (no thermals): 75.82,-0.64 75.82,20.83 69.47,27.18 25.65,27.18 19.81,21.34 19.81,-0.64
L_GPIO0  (via drill 0.3 pad 0.45)
  Top 0.127: U1.35 40.87,52.07 v43.69,52.07
  Top 0.406: R2.2 38.75,51.96 U1.35
  Route15 0.127: v43.69,52.07 54.36,52.07 55.88,50.55 62.74,50.55 67.77,55.58 JP4.4
L_GPIO1  (via drill 0.3 pad 0.45)
  Top 0.127: U1.36 43.07,50.69 v43.18,50.8
  Top 0.406: U1.36 38.86,50.69 37.34,49.17 37.34,44.7 35.15,42.52 R4.2
  Route15 0.127: v43.18,50.8 43.69,50.8 44.45,50.04 66.95,50.04 JP4.8
L_GPIO2  (via drill 0.3 pad 0.45)
  Top 0.127: U1.37 42.56,49.42 v42.67,49.53
  Top 0.406: U1.37 38.86,49.42 38.35,48.91 38.35,43.18 R6.2
  Route15 0.127: JP4.12 64.01,49.53 v42.67,49.53
L_GPIO8  (via drill 0.3 pad 0.45)
  Top 0.127: U1.45 42.27,39.26 v42.67,38.86
  Bottom 0.127: v42.67,38.86 52.32,29.21 77.88,29.21 JP5.2
L_GPIO9  (via drill 0.3 pad 0.45)
  Top 0.127: U1.46 42.53,37.99 v42.67,37.85
  Bottom 0.127: v42.67,37.85 52.07,28.45 76.1,28.45 JP5.1
L_GPIO10  (via drill 0.3 pad 0.45)
  Top 0.127: v61.21,53.09 58.69,53.09 U1.14
  Bottom 0.127: v61.21,53.09 55.12,53.09 54.36,52.32 54.36,35.56 56.13,33.78 74.05,33.78 JP5.8
L_GPIO11  (via drill 0.3 pad 0.45)
  Top 0.127: U1.13 61.07,51.96 v61.21,51.82
  Bottom 0.127: v61.21,51.82 56.13,51.82 55.12,50.8 55.12,35.81 56.39,34.54 72.27,34.54 JP5.9
L_GPIO12  (via drill 0.3 pad 0.45)
  Top 0.127: v61.21,48.01 58.69,48.01 U1.10
  Bottom 0.127: v61.21,48.01 56.9,48.01 55.88,46.99 55.88,36.07 56.64,35.31 70.5,35.31 JP5.10
L_GPIO13  (via drill 0.3 pad 0.45)
  Top 0.127: v61.21,46.74 58.69,46.74 U1.9
  Bottom 0.127: v61.21,46.74 57.4,46.74 56.64,45.97 56.64,36.58 57.15,36.07 68.72,36.07 JP5.11
N$1  (via drill 0.3 pad 0.45)
  Top 0.127: U2.7 47.96,72.69 v47.24,73.41 | R3.2 R2.1
  Route15 0.127: v47.24,73.41 47.24,66.55 31.95,51.26 R3.2
  other vias: 31.95,51.21
N$2  (via drill 0.3 pad 0.45)
  Top 0.127: U2.6 48.36,73.81 v48.01,74.17 | R5.2 R4.1
  Route15 0.127: R5.2 31.95,49.23 47.24,64.52 47.24,66.19 47.5,66.44 47.5,72.9 48.01,73.41 v48.01,74.17
  other vias: 31.95,45.42
N$3
  Top 1.016: JP1.15 JP1.16 10.79,50.13 14.73,50.13 F1.1
N$4
  Top 1.016: 9,55.24 JP1.11 JP1.9 | 9,55.24 10,55.24 | 10,55.24 JP1.12 JP1.10 10,57.78 | JP1.9 10,57.78 | JP1.9 9,57.78 9,55.24 | 10,55.24 10,57.78
N$7  (via drill 0.3 pad 0.45)
  Top 0.127: U2.5 48.76,73.65 v49.28,74.17 | R6.1 R7.2
  Route15 0.127: v49.28,74.17 49.28,59.69 44.32,54.74 31.95,42.37 R6.1
  other vias: 31.95,39.62
N$8  (2 unrouted)
  Top 0.102: 27.71,13.55 27.41,13.85 27.11,13.85 26.91,13.65 | 26.91,13.65 26.81,13.55 27.11,13.55 27.11,13.75 27.01,13.65 | 27.01,13.65 26.91,13.65 | 27.01,13.65 27.41,13.65 27.41,13.75 27.51,13.65 | 27.51,13.65 27.61,13.55 27.41,13.55 27.51,13.65 | 69.11,13.53 68.81,13.83 68.51,13.83 68.31,13.63 | 68.31,13.63 68.21,13.53 68.51,13.53 68.51,13.73 68.41,13.63 | 68.41,13.63 68.31,13.63 | 68.41,13.63 68.81,13.63 68.81,13.73 68.91,13.63 | 68.91,13.63 69.01,13.53 68.81,13.53 68.91,13.63
  Top 0.293: J1.RF 27.26,18.03 arc-90 29.8,20.57 66.12,20.57 arc-90 68.66,18.03 J2.RF
N$9  (via drill 0.3 pad 0.45)
  Top 0.127: U1.32 42.16,55.77 42.56,55.77 v42.93,56.13
  Bottom 0.127: v42.93,56.13 33.66,56.13 R1.1
  other vias: 31.85,54.33
N$10  (via drill 0.3 pad 0.45, 0.35 pad 0.8)
  Top 0.293: U1.23 v50.92,61.6 v50.93,61.59
  Route15 0.293: v50.93,61.59 50.93,56.64 51.69,55.88 56.13,55.88 60.45,60.2 74.07,60.2 R8.1
  other vias: 74.42,60.55
N$16  (via drill 0.3 pad 0.45)
  Top 0.127: U1.44 42.02,40.53 v42.67,39.88
  Bottom 0.127: v42.67,39.88 52.58,29.97 79.66,29.97 JP5.3
N$17  (via drill 0.3 pad 0.45)
  Top 0.127: U1.43 41.76,41.8 v42.67,40.89
  Bottom 0.127: v42.67,40.89 52.83,30.73 81.16,30.73 JP5.4
N$18  (via drill 0.3 pad 0.45)
  Top 0.127: U1.40 42.53,45.61 v42.67,45.47
  Bottom 0.127: v42.67,45.47 42.67,42.16 53.34,31.5 79.39,31.5 JP5.5
N$19  (via drill 0.3 pad 0.45)
  Top 0.127: U1.39 43.03,46.88 v43.18,46.74
  Bottom 0.127: v43.18,46.74 43.43,46.48 43.43,42.67 53.85,32.26 77.61,32.26 JP5.6
N$20  (via drill 0.3 pad 0.45)
  Top 0.127: U1.38 43.8,48.15 v43.94,48.01
  Bottom 0.127: v43.94,48.01 44.2,47.75 44.2,42.93 54.1,33.02 75.83,33.02 JP5.7
PGC_INT  (via drill 0.35 pad 0.8)
  Top 0.127: U1.30 43.07,58.31 v43.94,59.18
  Route15 0.127: v61.21,59.02 61.89,59.69 72.39,59.69 75.69,56.39 75.69,55.88 75.95,55.63 77.98,55.63 78.49,56.13 78.49,58.93 79.76,60.2 83.06,60.2 83.82,59.44 83.82,56.9 83.19,56.27 JP5.14
  Bottom 0.127: v43.94,59.18 47.05,59.18 47.29,59.42 60.81,59.42 v61.21,59.02
PGD_INT  (via drill 0.35 pad 0.8)
  Top 0.127: U1.31 42.82,57.04 v43.43,57.66
  Route15 0.127: v61.25,57.37 65.56,57.37 65.79,57.15 73.41,57.15 75.44,55.12 78.74,55.12 78.99,55.37 78.99,56.9 80.91,58.81 JP5.15
  Bottom 0.127: v43.43,57.66 60.96,57.66 v61.25,57.37
RX  (via drill 0.3 pad 0.45)
  Top 0.127: U1.6 v61.21,43.07
  Route15 0.127: v61.21,43.07 55.48,43.07 55.12,43.43 39.88,43.43 34.29,37.85 30.48,37.85 28.45,39.88 | 28.45,39.88 JP3.6 | 28.45,39.88 28.45,45.72 | 28.45,45.72 27.18,46.99 JP3.10 | 28.45,45.72 28.45,50.04 JP3.14
RX0
  Top 0.406: JP3.13 11.81,40.01 JP1.24
RX1
  Top 0.406: JP3.9 11.81,34.92 JP1.28
RX2
  Top 0.406: JP3.5 11.81,29.84 JP1.32
TX  (via drill 0.3 pad 0.45)
  Top 0.127: U1.7 61.11,44.34 v61.21,44.45 | v29.21,42.16 JP3.4 | v29.21,42.16 26.92,44.45 JP3.8 | v29.21,42.16 29.21,46.74 JP3.12
  Route15 0.127: v29.21,42.16 29.21,40.13 30.73,38.61 34.04,38.61 39.37,43.94 54.86,43.94 55.37,44.45 v61.21,44.45
TX0
  Top 0.406: JP3.11 11.81,37.47 JP1.26
TX1
  Top 0.406: JP3.7 11.81,32.38 JP1.30
TX2
  Top 0.406: JP3.3 11.81,27.3 JP1.34
UARTCTS  (via drill 0.3 pad 0.45)
  Top 0.127: v60.96,39.37 60.85,39.26 U1.3
  Bottom 0.127: v60.96,39.37 57.91,39.37 57.4,38.86 57.4,37.59 58.17,36.83 66.94,36.83 JP5.12
UARTRTS  (via drill 0.3 pad 0.45)
  Top 0.127: v60.96,37.59 60.56,37.99 U1.2
  Bottom 0.127: JP5.13 65.16,37.59 v60.96,37.59

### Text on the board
tPlace: JLCJLCJLCJLC | BOARD # / 1 2 3 4 | RAD | REV B
tNames: U3 | GND | PGD | GND | PDC | External | VCC | IO0 | RTS | GND | RX0 | CTS | IO1 | VCC | TX0 | IO13 | GND | IO12 | RX1 | IO2 | TX1 | IO11 | IO10 | RX2 | IO9 | TX2 | IO8 | GND | IO7 | IO6 | IO5 | IO4 | IO3 | JP5

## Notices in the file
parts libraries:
SparkFun-PowerSymbols: Licensing: Creative Commons ShareAlike 4.0 International - https://creativecommons.org/licenses/by-sa/4.0
